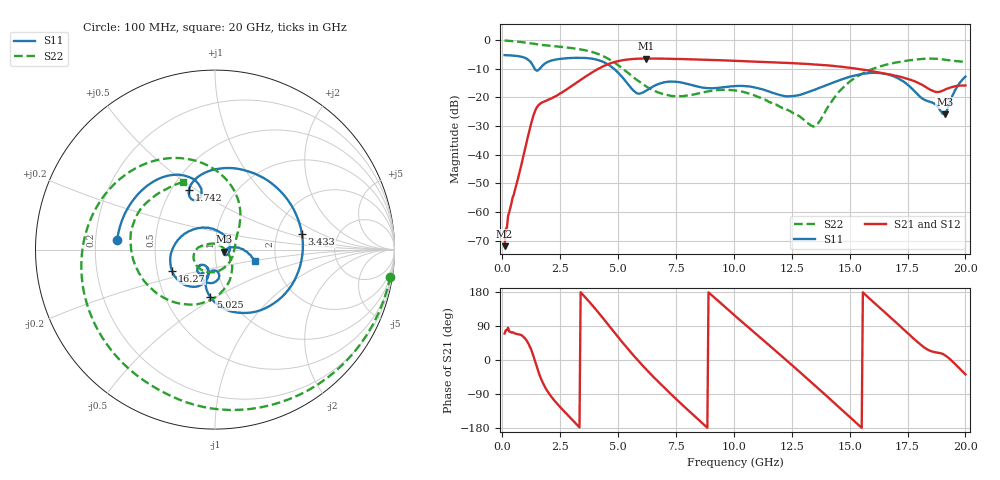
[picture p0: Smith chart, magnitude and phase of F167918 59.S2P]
!  2-Port S-parameters saved by WinCal
! VAR MeasName=S-Parameters (CALIBRATED_DATA) read from VNA (N5242A)
! VAR MeasDate=2016-11-22 10:27:44
! VAR NAME=F167918 59
! VAR FILENAME=F167918 59.S2P
! VAR DATE=2016-11-22 10:27:44
! VAR PHYS_PORTS=1,2
# Hz S DB R 50
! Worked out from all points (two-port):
!   401 points, 100 MHz to 20 GHz, reference 50 ohm
!   highest |S21| = -6.41 dB at 6.219 GHz (marker M1); lowest = -72.0 dB at 100 MHz (marker M2)
!   |S21| within 3 dB of the highest: 4.288 GHz to 14.77 GHz (10.48 GHz wide, 110 % of centre)
!   lowest |S11| = -25.9 dB at 19.1 GHz (marker M3), VSWR 1.11, Z = 55.2 - j1.22 ohm
!   |S11| at or under -10 dB: 1.404 GHz to 1.614 GHz (210.2 MHz wide, 13.9 % of centre); 4.822 GHz to end of sweep
!   |S22| runs from -30.2 to -0.1 dB; largest |S21 - S12| = 0.0038
!   S11 on the Smith chart (normalised r, x): 100 MHz: 0.29, +0.04; 1.742 GHz: 0.61, +0.46; 3.433 GHz: 2.77, +0.64; 5.025 GHz: 0.83, -0.47; 16.27 GHz: 0.60, -0.15; 20 GHz: 1.55, -0.21
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1e8  -5.23 174.6  -71.96 69.9  -70.36 87.0  -0.10 -8.8
8.96e8  -5.93 129.2  -40.99 62.1  -41.06 62.3  -0.72 -70.7
1.3935e9  -9.88 103.5  -25.20 1.1  -25.21 1.1  -1.33 -103.8
1.74175e9  -8.85 113.8  -21.68 -59.1  -21.67 -59.2  -1.69 -123.4
2.53775e9  -6.51 68.2  -18.44 -126.8  -18.45 -126.9  -2.33 -164.0
3.43325e9  -6.16 10.2  -13.59 175.5  -13.60 175.7  -3.29 153.1
4.279e9  -7.32 -49.4  -9.44 115.8  -9.41 115.8  -5.28 110.5
5.02525e9  -11.52 -95.9  -7.26 58.7  -7.25 58.6  -8.87 74.5
5.7715e9  -18.34 -99.4  -6.48 4.7  -6.47 4.6  -13.65 48.2
6.21925e9  -17.60 -81.3  -6.41 -25.0  -6.41 -25.1  -16.23 35.8
6.7665e9  -15.25 -86.3  -6.43 -59.3  -6.43 -59.4  -18.37 19.0
7.61225e9  -14.63 -108.3  -6.56 -109.1  -6.55 -109.1  -19.57 -21.9
8.5575e9  -16.43 -119.0  -6.75 -162.3  -6.73 -162.3  -18.45 -78.6
1.005e10  -16.01 -121.2  -7.22 116.7  -7.21 116.7  -17.56 -149.9
1.189075e10  -18.93 -130.9  -7.82 19.5  -7.80 19.4  -22.86 163.1
1.338325e10  -17.64 -105.2  -8.41 -60.9  -8.37 -60.8  -29.92 83.0
1.497525e10  -12.87 -115.8  -9.63 -148.6  -9.58 -149.0  -14.68 -63.0
1.626875e10  -11.45 -153.9  -11.26 139.8  -11.27 139.7  -9.27 -117.4
1.67165e10  -12.12 -173.6  -11.92 115.3  -12.01 115.0  -8.30 -133.7
1.805975e10  -19.93 75.1  -15.28 41.0  -15.27 41.4  -6.60 180.0
1.91045e10  -25.86 -12.5  -17.36 13.1  -17.28 13.2  -6.82 142.0
2e10  -12.75 -16.5  -15.81 -37.9  -15.73 -37.6  -7.62 115.7
